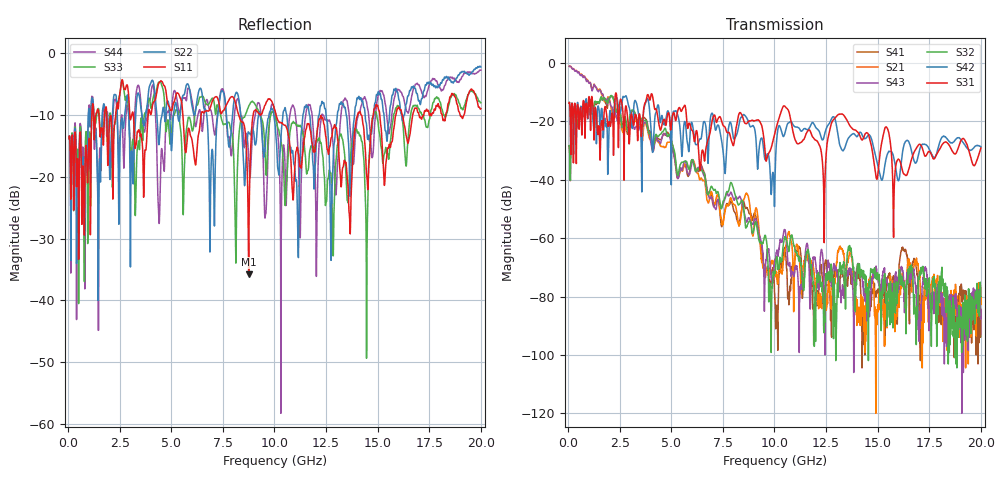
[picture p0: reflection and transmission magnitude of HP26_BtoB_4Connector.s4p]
# MHz S MA R 50.00
! FREQ  S11  S12  S13  S14
!  S21  S22  S23  S24
!  S31  S32  S33  S34
!  S41  S42  S43  S44
!  MAG  ANG  MAG  ANG  MAG  ANG  MAG  ANG
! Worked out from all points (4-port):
!   1996 points, 50 MHz to 20 GHz, reference 50 ohm
!   strongest paths, dB at 50 MHz, 5.04 GHz, 10.03 GHz, 15.02 GHz, 20 GHz:
!     S31: -13.8, -18.7, -23.8, -37.3, -29.2
!     S42: -13.8, -21.3, -38.4, -35.4, -28.7
!     S32: -28.3, -27.6, -71.3, -73.6, -80.0
!     S43: -1.1, -29.1, -68.0, -74.8, -84.7
!     S21: -1.1, -27.6, -69.6, -82.7, -80.2
!     S41: -28.4, -27.7, -82.6, -77.7, -84.4
!   lowest |S11| = -35.7 dB at 8.75 GHz (marker M1), VSWR 1.03, Z = 48.5 - j0.693 ohm
!   |S11| at or under -10 dB: start of sweep to 1.15 GHz; 5.56 GHz to 6.446 GHz (885.8 MHz wide, 14.8 % of centre); 10.08 GHz to 14.03 GHz (3.954 GHz wide, 32.8 % of centre)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
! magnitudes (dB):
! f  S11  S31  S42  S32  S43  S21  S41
! 50 MHz  -13.9  -13.8  -13.8  -28.3  -1.1  -1.1  -28.4
! 2.11 GHz  -11.9  -17.6  -20.4  -11.2  -14.9  -16.2  -11.6
! 8.75 GHz  -35.7  -20.0  -20.6  -54.4  -53.0  -46.3  -50.9
! 10.09 GHz  -10.2  -22.1  -27.8  -67.2  -65.0  -73.0  -84.2
! 12.4 GHz  -11.6  -51.5  -25.2  -87.5  -80.0  -77.0  -73.7
! 14.46 GHz  -19.7  -23.9  -25.6  -76.2  -83.0  -80.9  -80.6
! 20 GHz  -9.0  -29.2  -28.7  -80.0  -84.7  -80.2  -84.4
